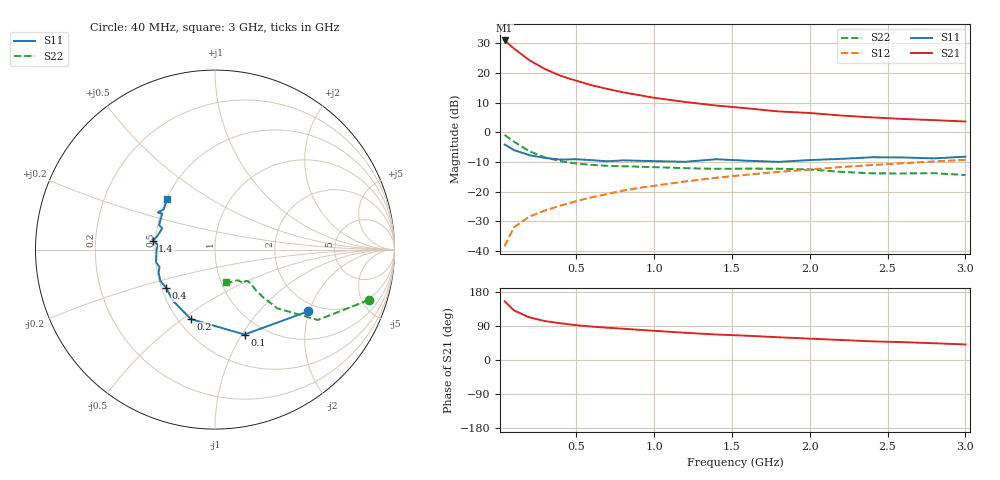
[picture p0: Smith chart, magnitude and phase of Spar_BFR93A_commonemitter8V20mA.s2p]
! Filename:  BFR93AG.S2P  Version:  2.0
! NXP part #: BFR93A  Date: May 1990
! Bias condition: Vce=8V, Ic=20mA
#  MHz  S  MA  R  50
! Freq  S11  S21  S12  S22  !GUM [dB]
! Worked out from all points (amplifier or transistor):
!   21 points, 40 MHz to 3 GHz, reference 50 ohm
!   highest |S21| = 31.0 dB at 40 MHz (marker M1)
!   |S21| within 3 dB of that: start of sweep to 106.8 MHz
!   unconditionally stable (mu >= 1): 691 MHz to 732 MHz; 847.8 MHz to 2.849 GHz
!   at 300 MHz: K = 0.81, MSG = 23.8 dB, |S12| = -26.4 dB
!   at 1 GHz: K = 1.03, MAG = 13.8 dB, |S12| = -18.1 dB
!   at 3 GHz: K = 0.99, MSG = 6.5 dB, |S12| = -9.3 dB
!   S11 on the Smith chart (normalised r, x): 40 MHz: 1.75, -1.97; 100 MHz: 0.81, -1.03; 200 MHz: 0.58, -0.54; 400 MHz: 0.53, -0.26; 1.4 GHz: 0.48, +0.06; 3 GHz: 0.50, +0.33
40  0.623 -33.5  35.36 154.9  0.012 76.1  0.901 -18.2
100  0.501 -70.8  25.82 130.9  0.025 62.7  0.694 -34.4
200  0.41 -109.3  16.36 112.3  0.038 62.0  0.477 -43.3
300  0.369 -129.1  11.63 102.7  0.048 63.3  0.377 -44.7
400  0.346 -141.8  8.956 96.9  0.058 65.8  0.325 -44.9
500  0.351 -150.3  7.403 91.8  0.069 66.7  0.297 -44.2
600  0.339 -158.0  6.202 88.2  0.08 69.2  0.281 -43.8
700  0.324 -162.5  5.386 85.2  0.091 69.8  0.272 -44.1
800  0.336 -168.1  4.723 82.5  0.104 70.2  0.267 -43.5
900  0.331 -171.1  4.25 79.8  0.115 70.7  0.263 -43.9
1000  0.326 179.9  3.818 77.1  0.125 70.7  0.258 -43.7
1200  0.318 175.4  3.245 71.8  0.148 70.5  0.248 -44.7
1400  0.351 171.7  2.823 67.3  0.171 69.8  0.242 -47.1
1600  0.331 167.2  2.53 64.0  0.193 69.3  0.244 -48.5
1800  0.317 158.1  2.248 60.0  0.215 68.1  0.243 -50.2
2000  0.34 156.3  2.114 56.4  0.235 67.2  0.236 -50.7
2200  0.356 145.7  1.918 52.8  0.259 66.7  0.215 -52.8
2400  0.379 147.0  1.784 49.3  0.28 64.9  0.203 -59.2
2600  0.376 145.8  1.677 47.1  0.301 63.7  0.202 -66.0
2800  0.363 141.8  1.601 44.2  0.322 62.7  0.204 -68.6
3000  0.388 133.5  1.519 41.0  0.342 60.9  0.19 -70.5
